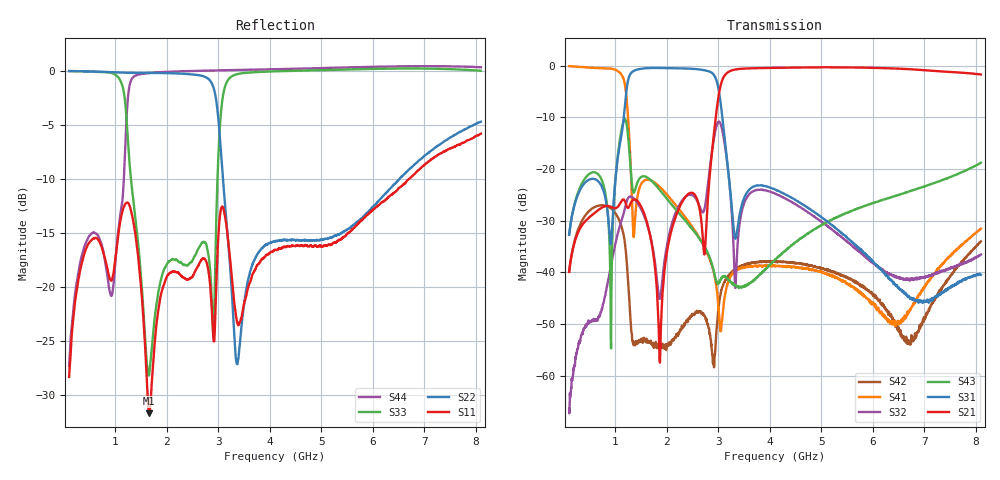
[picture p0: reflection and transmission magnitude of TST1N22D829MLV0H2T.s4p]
# MHZ S RI R 50
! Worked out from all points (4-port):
!   1601 points, 100 MHz to 8.1 GHz, reference 50 ohm
!   strongest paths, dB at 100 MHz, 2.1 GHz, 4.1 GHz, 6.1 GHz, 8.1 GHz:
!     S21: -39.9, -31.4, -0.4, -0.4, -1.7
!     S31: -32.7, -0.5, -23.9, -38.9, -40.4
!     S43: -32.7, -27.0, -37.5, -26.3, -18.8
!     S32: -66.3, -30.4, -24.7, -38.9, -36.5
!     S41: -0.1, -26.1, -38.7, -47.2, -31.5
!     S42: -39.9, -53.2, -37.9, -45.3, -34.0
!   lowest |S11| = -31.7 dB at 1.655 GHz (marker M1), VSWR 1.05, Z = 52.1 - j1.57 ohm
!   |S11| at or under -10 dB: start of sweep to 6.699 GHz
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100  -0.00368 -0.0381  0.00168 0.0101  0.00419 0.0227  0.9615 -0.2437
     0.0018 0.00996  0.9682 -0.2563  -0.000123 0.000466  0.00373 0.00945
     0.00428 0.0228  -0.000183 0.000446  0.9898 -0.1506  0.00594 0.0224
     0.9597 -0.2442  0.00372 0.00946  0.00589 0.0224  0.00245 -0.0428
970  -0.0759 0.0918  0.0296 0.0295  -0.0422 0.0296  -0.9015 -0.201
     0.0298 0.0297  -0.5283 -0.8354  -0.0146 0.00697  -0.0325 -0.0217
     -0.0422 0.0297  -0.0146 0.00709  -0.2289 -0.945  3.69e-05 0.0484
     -0.9021 -0.2018  -0.0325 -0.0218  -7.71e-05 0.0484  0.0464 0.0963
1655  0.0211 -0.015  0.0253 0.00128  0.9429 0.1211  -0.0738 0.0271
      0.0252 0.00138  -0.9786 -0.0715  0.024 0.00729  -0.00206 0.000613
      0.9419 0.1217  0.024 0.00716  -0.014 -0.0366  0.0306 -0.0745
      -0.0739 0.0272  -0.00209 0.000552  0.0307 -0.0747  -0.1194 -0.9733
1865  -0.0774 -0.0402  -0.00066 -0.00124  0.8859 -0.3475  -0.0483 0.0464
      -0.000489 -0.00125  -0.9654 0.1733  0.00184 0.00518  -0.00116 0.00154
      0.8854 -0.3476  0.00201 0.00522  0.0363 -0.0966  0.00394 -0.0623
      -0.0483 0.0463  -0.00117 0.00158  0.00397 -0.0624  -0.3526 -0.9242
2855  0.0236 -0.0882  0.0625 -0.0968  -0.8475 -0.1722  0.0105 0.00672
      0.0631 -0.0973  0.4651 0.7616  -0.00899 0.1242  0.00202 0.000679
      -0.8467 -0.1735  -0.00903 0.1235  0.0779 -0.0705  -0.0121 -0.00452
      0.0104 0.0067  0.00203 0.000861  -0.012 -0.00447  -0.7311 -0.692
3330  -0.0229 -0.0737  -0.8886 0.2344  -0.0211 0.00337  0.000973 0.0104
      -0.8891 0.2359  -0.000421 -0.0499  0.00651 -0.00247  -0.00543 0.00935
      -0.0209 0.00348  0.00663 -0.00251  0.7294 -0.6298  -0.00739 0.000353
      0.0011 0.0103  -0.00537 0.0092  -0.00753 0.00034  -0.7901 -0.6331
8100  -0.1372 -0.4944  0.8123 -0.1023  0.00224 -0.00933  -0.024 0.011
      0.8172 -0.1016  -0.0188 -0.5827  -0.00263 0.0147  -0.0197 0.00297
      0.00214 -0.00927  -0.00243 0.0147  -0.9645 0.2814  0.00397 0.1143
      -0.0242 0.0108  -0.0198 0.00299  0.00326 0.1153  -0.991 -0.325
